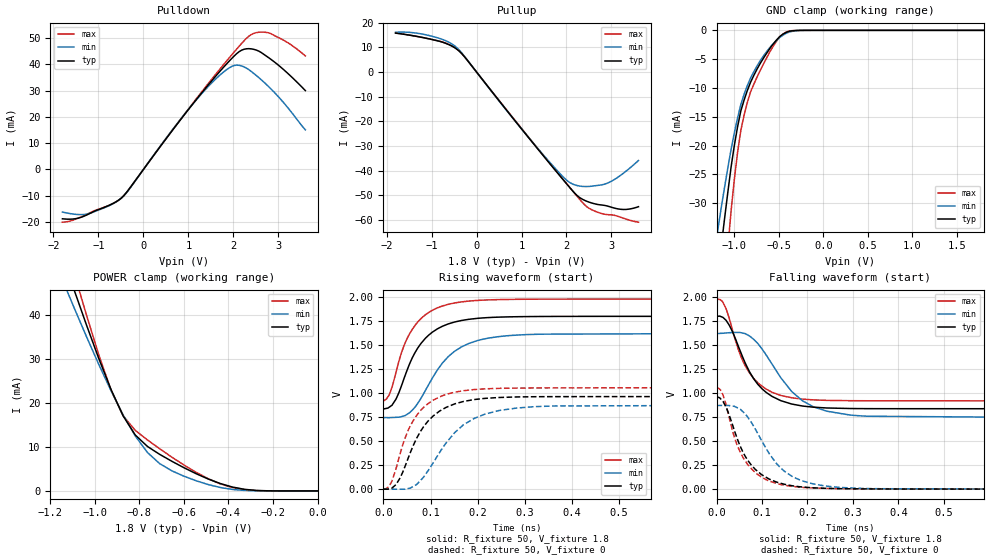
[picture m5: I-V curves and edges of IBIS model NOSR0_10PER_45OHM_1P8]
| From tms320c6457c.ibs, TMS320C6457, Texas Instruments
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|   Model Cell NOSR0_10PER_45OHM_1P8
|NOSR0_10PER_45OHM_1P8
[Model]   NOSR0_10PER_45OHM_1P8
Model_type   3-state
Polarity   Non-Inverting
Enable   Active-Low
Cref =  15.0000pF
Rref =  100.0000M
Vref =  0V
Vmeas =  0.9
C_comp   1.89p   1.72p   2.18p
[Model Spec]
Rref 50 NA NA
Vref 0.9 0.81 0.99
[Temperature Range]   25   125   -40
[Voltage Range]   1.8   1.62   1.98
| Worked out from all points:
|   slope of the pulldown table from 0 to 0.27 V, typ, clamps not added: 42.8 ohm
|   slope of the pullup table from 0 to 0.27 V, typ, clamps not added: 43 ohm
|   GND clamp passes 1 mA (typ) near -0.48 V on its own axis
|   POWER clamp passes 1 mA (typ) near -0.39 V on its own axis
|   rising waveform, R_fixture 50, V_fixture 1.8: 20-80 % time 62.1ps typ, 77.6ps min, 55.8ps max; typ from 0.838 V to 1.8 V
|   rising waveform, R_fixture 50, V_fixture 0: 20-80 % time 65.8ps typ, 86.5ps min, 57.5ps max; typ from 0.001 V to 0.965 V
|   falling waveform, R_fixture 50, V_fixture 1.8: 20-80 % time 65.8ps typ, 86.4ps min, 57.5ps max; typ from 1.8 V to 0.838 V
|   falling waveform, R_fixture 50, V_fixture 0: 20-80 % time 60.6ps typ, 76.7ps min, 54.4ps max; typ from 0.965 V to 0.001 V
| Nom Voltages:
|   BIAS2=0.9, BIASFET=0, VDD=1.1, VDDS=1.8, BUS_BIAS1=0, BUS_BIAS3=0,
|   VSS=0, VSSS=0
| Min Voltages:
|   BIAS2=0.81, BIASFET=0, VDD=0.99, VDDS=1.62, BUS_BIAS1=0, BUS_BIAS3=0,
|   VSS=0, VSSS=0
| Max Voltages:
|   BIAS2=0.99, BIASFET=0, VDD=1.21, VDDS=1.98, BUS_BIAS1=0, BUS_BIAS3=0,
|   VSS=0, VSSS=0
[POWER_clamp]
|   voltage   I(typ)   I(min)   I(max)
-1.8V     156mA      133.5mA    181.7mA
-1.127V   50.87mA    45.88mA    55.74mA
-1.109V   48.19mA    43.68mA    52.51mA
-1.073V   42.88mA    39.33mA    46.15mA
-1.055V   40.27mA    37.18mA    43.01mA
-927.3mV  23.11mA    22.83mA    22.99mA
-872.7mV  17.08mA    17.31mA    17.08mA
-818.2mV  12.73mA    12.5mA     13.8mA
-763.6mV  10.13mA    8.758mA    11.61mA
-600mV    5.297mA    3.359mA    5.911mA
-381.8mV  881.1uA    334.9uA    769uA
0V        130.3nA    147.3nA    381.2nA
[Pulldown]
|   voltage   I(typ)   I(min)   I(max)
-1.8V     -18.75mA   -16.19mA   -20.05mA
-1.527V   -18.77mA   -17.02mA   -19.04mA
-1.255V   -17.27mA   -16.96mA   -17.01mA
-490.9mV  -10.86mA   -10.92mA   -10.93mA
1.2V      27.09mA    26.95mA    27.4mA
1.691V    37.13mA    35.74mA    37.97mA
2.018V    43.17mA    39.55mA    44.69mA
2.291V    45.9mA     38.54mA    49.87mA
2.455V    45.69mA    36.51mA    51.76mA
2.673V    43.84mA    33.31mA    52.23mA
3.164V    37.26mA    24.47mA    48.7mA
3.6V      30mA       15.08mA    43.19mA
[Pullup]
|   voltage   I(typ)   I(min)   I(max)
-1.8V     15.73mA    16.1mA     15.85mA
-1.364V   14.54mA    15.81mA    14.51mA
-927.3mV  12.89mA    14.16mA    12.9mA
-600mV    10.96mA    11.91mA    11.06mA
-381.8mV  8.4mA      8.842mA    8.439mA
1.309V    -29.99mA   -29.83mA   -29.82mA
1.909V    -43.26mA   -42.17mA   -43.16mA
2.127V    -47.95mA   -45.3mA    -47.94mA
2.455V    -52.38mA   -46.38mA   -54.61mA
2.891V    -54.19mA   -45.14mA   -57.73mA
3.273V    -55.67mA   -40.88mA   -59.26mA
3.6V      -54.55mA   -35.84mA   -60.82mA
[GND_clamp]
|   voltage   I(typ)   I(min)   I(max)
-1.8V     -137.1mA   -107.1mA   -189.7mA
-1.182V   -42.18mA   -34.28mA   -58.62mA
-1.109V   -32.61mA   -27.18mA   -44.51mA
-1.073V   -28.08mA   -23.86mA   -37.8mA
-1.036V   -23.72mA   -20.65mA   -31.33mA
-963.6mV  -16.74mA   -15.21mA   -21.21mA
-927.3mV  -13.99mA   -12.88mA   -17.38mA
-854.5mV  -10.47mA   -9.599mA   -12.54mA
-781.8mV  -7.837mA   -7.198mA   -9.373mA
-600mV    -3.116mA   -2.961mA   -3.703mA
-418.2mV  -354.7uA   -522.3uA   -297.6uA
1.8V      130.3nA    2.912uA    201.9nA
[Ramp]
| variable   typ   min   max
dV/dt_f 0.48421492/51.530415p 0.44231855/68.570024p 0.53157772/44.934746p
dV/dt_r 0.48481069/51.640901p 0.43888484/67.415723p   0.530125/45.102173p
R_load = 50
[Rising Waveform]
R_fixture = 50
V_fixture = 1.8
V_fixture_min = 1.62
V_fixture_max = 1.98
|   time   V(typ)   V(min)   V(max)
0s        838mV      747.5mV    919.3mV
12.3ps    853.7mV    744.8mV    981.6mV
26.9ps    939.1mV    748.2mV    1.22V
44.1ps    1.158V     763.2mV    1.499V
63.5ps    1.389V     834.8mV    1.681V
96.6ps    1.606V     1.094V     1.842V
150.5ps   1.74V      1.434V     1.939V
200.4ps   1.779V     1.549V     1.966V
305.9ps   1.797V     1.61V      1.978V
1.185ns   1.8V       1.62V      1.98V
[Rising Waveform]
R_fixture = 50
V_fixture = 0
V_fixture_min = 0
V_fixture_max = 0
|   time   V(typ)   V(min)   V(max)
0s        660.5uV    0V         138.2uV
12.47ps   4.004mV    0V         32.48mV
26.9ps    48.61mV    0V         215mV
46.9ps    249.9mV    1.029mV    544mV
70.9ps    533.8mV    50.12mV    769.6mV
105.1ps   760.2mV    270.2mV    924.8mV
151.4ps   888.4mV    589.4mV    1.01V
215.4ps   945.4mV    781.4mV    1.045V
317.4ps   962.5mV    857.8mV    1.054V
1.185ns   964.6mV    870.8mV    1.057V
[Falling Waveform]
R_fixture = 50
V_fixture = 1.8
V_fixture_min = 1.62
V_fixture_max = 1.98
|   time   V(typ)   V(min)   V(max)
0s        1.8V       1.62V      1.98V
14.1ps    1.789V     1.624V     1.946V
28.1ps    1.707V     1.629V     1.776V
51.3ps    1.449V     1.632V     1.41V
81.7ps    1.151V     1.561V     1.154V
122.3ps   966mV      1.302V     1.009V
165.3ps   887.1mV    1.018V     952.4mV
213ps     854.2mV    858.4mV    930.3mV
320.1ps   839.3mV    762.9mV    921.2mV
1.185ns   838.2mV    748.4mV    920mV
[Falling Waveform]
R_fixture = 50
V_fixture = 0
V_fixture_min = 0
V_fixture_max = 0
|   time   V(typ)   V(min)   V(max)
0s        964.6mV    872.2mV    1.057V
8.566ps   943.7mV    872.2mV    1.035V
21.1ps    854.3mV    872.2mV    877mV
45.1ps    532.8mV    849.9mV    463.5mV
69ps      298.8mV    748.6mV    254.6mV
99ps      152.4mV    508.5mV    126.1mV
149.7ps   51.08mV    186.2mV    41.18mV
211ps     15.37mV    57.92mV    13.5mV
320.2ps   3.625mV    8.289mV    4.167mV
1.185ns   994.8uV    1.087mV    623.9uV
